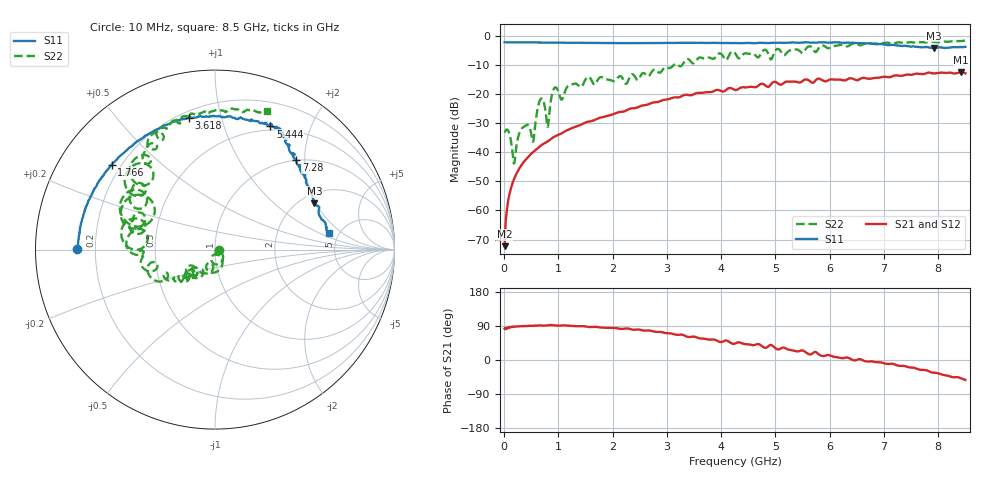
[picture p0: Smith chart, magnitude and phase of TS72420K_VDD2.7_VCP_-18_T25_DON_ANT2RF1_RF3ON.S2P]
!Agilent Technologies,E5071C,MY46417908,A.11.23
!Date: Thu Oct 03 16:41:16 2019
!Data & Calibration Information:
!Freq	S11:SOLT2(ON)	S21:SOLT2(ON)	S12:SOLT2(ON)	S22:SOLT2(ON)
!PortZ  Port1:50+j0  Port2:50+j0
!Above PortZ is port z conversion or system Z0 setting when saving the data.
!When reading, reference impedance value at option line is always used.
# Hz S dB R 50
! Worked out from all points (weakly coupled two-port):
!   1601 points, 10 MHz to 8.5 GHz, reference 50 ohm
!   highest |S21| = -12.57 dB at 8.42 GHz (marker M1); lowest = -72.2 dB at 10 MHz (marker M2)
!   lowest |S11| = -4.3 dB at 7.922 GHz (marker M3), VSWR 4.14, Z = 118 + j97.2 ohm
!   |S11| at or under -10 dB: nowhere
!   |S22| runs from -43.9 to -1.7 dB; largest |S21 - S12| = 0.0031
!   S11 on the Smith chart (normalised r, x): 10 MHz: 0.13, +0.00; 1.766 GHz: 0.16, +0.35; 3.618 GHz: 0.24, +0.79; 5.444 GHz: 0.46, +1.45; 7.28 GHz: 1.00, +1.82; 8.5 GHz: 4.11, +1.32
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1e7  -2.31 179.9  -72.23 82.8  -73.45 80.2  -33.28 -0.2
8.42875e7  -2.33 178.1  -55.70 85.4  -55.78 85.4  -32.92 -38.8
1.851062e8  -2.36 175.7  -49.10 87.8  -49.27 87.8  -43.87 -38.1
3.177625e8  -2.38 172.6  -44.54 89.3  -44.56 89.0  -32.06 -41.5
5.300125e8  -2.39 168.1  -40.04 90.1  -40.09 89.9  -36.43 -60.5
6.838938e8  -2.41 164.6  -37.65 91.1  -37.69 90.9  -21.57 -76.4
8.059375e8  -2.41 162.0  -36.26 91.5  -36.31 91.4  -31.34 -80.0
9.385938e8  -2.44 159.1  -34.56 91.3  -34.59 91.0  -17.78 -94.1
1.060638e9  -2.47 156.5  -33.53 91.2  -33.56 91.0  -22.01 -108.6
1.203906e9  -2.47 153.2  -32.13 90.3  -32.15 90.1  -16.97 -110.3
1.426769e9  -2.52 148.4  -30.50 89.4  -30.50 89.2  -17.54 -121.0
1.766369e9  -2.56 140.6  -28.20 86.0  -28.18 85.9  -14.35 -131.1
2.843538e9  -2.57 116.5  -22.74 74.3  -22.69 74.3  -12.62 -143.5
3.61825e9  -2.49 101.3  -19.68 56.9  -19.67 57.1  -7.54 -169.8
4.255e9  -2.57 88.1  -18.67 43.5  -18.66 43.6  -6.02 160.2
5.4436e9  -2.47 65.8  -16.11 23.6  -16.08 23.7  -5.27 137.8
5.671769e9  -2.42 63.4  -16.14 16.2  -16.14 16.4  -4.12 129.6
7.088538e9  -3.30 50.7  -14.30 -10.6  -14.34 -10.6  -2.54 106.1
7.279562e9  -3.45 47.7  -13.77 -15.3  -13.80 -15.8  -2.34 103.2
7.921619e9  -4.28 24.9  -13.02 -33.5  -12.92 -33.5  -2.21 86.6
8.420406e9  -3.94 11.1  -12.57 -48.6  -12.59 -48.7  -1.89 72.0
8.5e9  -3.87 8.5  -12.96 -52.6  -13.03 -52.5  -1.69 69.2
